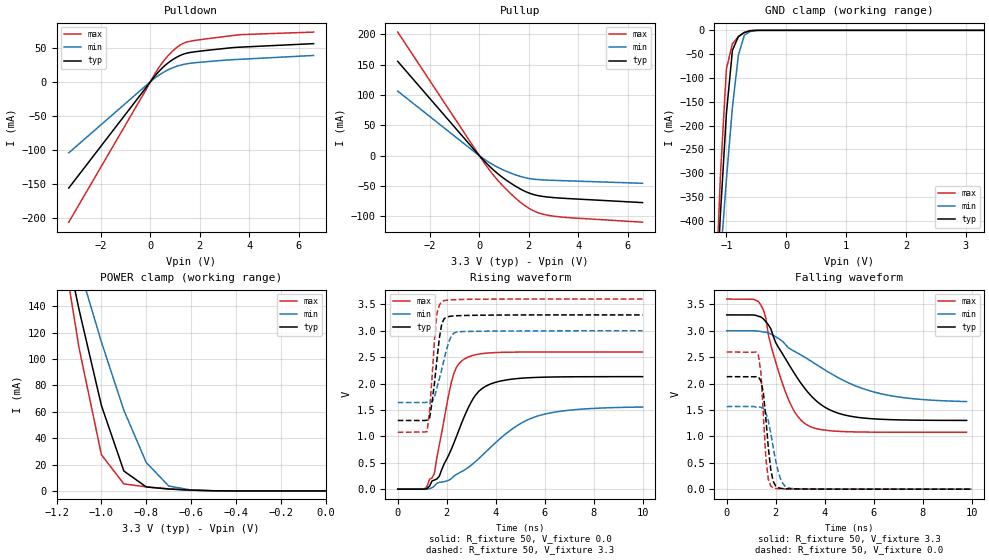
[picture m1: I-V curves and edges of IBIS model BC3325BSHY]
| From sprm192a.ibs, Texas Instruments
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[Model]   BC3325BSHY
Model_type   I/O
Vinh = 2.00
Vinl = 0.80
Enable   Active-Low
Polarity   Non-Inverting
| signals   A, GZ, Y
Vmeas = 1.5
|   typ   min   max
C_comp   1.4592p   1.4336p   1.5063p
|   typ   min   max
[Temperature Range]   25   -40   125
|   typ   min   max
[Voltage Range]   3.30V   3.00V   3.60V
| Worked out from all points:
|   slope of the pulldown table from 0 to 0.495 V, typ, clamps not added: 24 ohm
|   slope of the pullup table from 0 to 0.495 V, typ, clamps not added: 23.8 ohm
|   GND clamp passes 1 mA (typ) near -0.60 V on its own axis
|   POWER clamp passes 1 mA (typ) near -0.65 V on its own axis
|   rising waveform, R_fixture 50, V_fixture 0.0: 20-80 % time 1.22ns typ, 2.5ns min, 651ps max; typ from 0 V to 2.13 V
|   falling waveform, R_fixture 50, V_fixture 3.3: 20-80 % time 1.69ns typ, 3.01ns min, 992ps max; typ from 3.3 V to 1.3 V
|   rising waveform, R_fixture 50, V_fixture 3.3: 20-80 % time 298ps typ, 453ps min, 241ps max; typ from 1.3 V to 3.3 V
|   falling waveform, R_fixture 50, V_fixture 0.0: 20-80 % time 263ps typ, 401ps min, 201ps max; typ from 2.13 V to 0 V
[Pulldown]
|   Voltage   I(typ)   I(min)   I(max)
-3.3V     -155.6mA   -104.1mA   -205.7mA
200mV     9.245mA    5.867mA    12.7mA
600mV     24.13mA    15.28mA    33.3mA
800mV     29.87mA    18.87mA    41.37mA
1.1V      36.63mA    23.02mA    51.08mA
1.3V      39.97mA    25.04mA    55.82mA
1.6V      42.83mA    27mA       59.29mA
3.5V      50.44mA    32.65mA    68.4mA
6.6V      55.85mA    38.51mA    72.74mA
[GND_clamp]
|   Voltage   I(typ)   I(min)   I(max)
-3.3V     -6.256A    -4.713A    -8.133A
-1.2V     -625.1mA   -657.9mA   -612.5mA
-1.1V     -386.1mA   -480.8mA   -304.3mA
-1V       -174.5mA   -312.6mA   -80.61mA
-900mV    -42.06mA   -162mA     -28.39mA
-800mV    -12.94mA   -52.09mA   -13.55mA
-700mV    -4.666mA   -10.15mA   -3.941mA
-600mV    -901.9uA   -2.273mA   -447.8uA
-400mV    -4.618uA   -49.07uA   -472nA
3.3V      133.2pA    1.904uA    0A
[Pullup]
|   Voltage   I(typ)   I(min)   I(max)
-3.3V     155.5mA    106.5mA    203.8mA
-200mV    9.305mA    6.232mA    12.42mA
300mV     -13.07mA   -8.545mA   -17.75mA
600mV     -24.68mA   -16mA      -33.64mA
900mV     -34.78mA   -22.33mA   -47.63mA
1.4V      -48.81mA   -30.78mA   -67.77mA
1.7V      -55.89mA   -34.78mA   -78.18mA
2V        -61.53mA   -37.68mA   -86.7mA
2.3V      -65.31mA   -39.22mA   -93.01mA
2.9V      -68.84mA   -40.61mA   -99.22mA
3.7V      -71.03mA   -41.73mA   -102.5mA
6.6V      -77.47mA   -45.64mA   -109.8mA
[POWER_clamp]
|   Voltage   I(typ)   I(min)   I(max)
-3.3V     2.13A      1.607A     2.766A
-1.2V     219.2mA    230.5mA    214.4mA
-1.1V     137.7mA    170.3mA    108.7mA
-1V       64.77mA    112.9mA    27.43mA
-900mV    15.1mA     61.17mA    5.337mA
-800mV    3.01mA     21.5mA     3.051mA
-700mV    1.426mA    3.717mA    1.578mA
-600mV    596.1uA    671uA      553.1uA
0V        399.7pA    9.948nA    88.82pA
[Ramp]
|   I(typ)   I(min)   I(max)
dV/dt_r   1.278/1.224n   0.933/2.499n   1.559/0.649n
dV/dt_f   1.199/1.689n   0.806/3.020n   1.513/0.992n
[Rising Waveform]
R_fixture = 50
V_fixture = 0.0
|  pu_on
|  TIME   V(typ)   V(min)   V(max)
0s        3nV        16nV       2nV
1.1ns     -133.6uV   -280.8uV   2.733mV
1.4ns     153.6mV    26.81mV    210.9mV
1.5ns     172.7mV    58.73mV    301.8mV
2.2ns     766.4mV    203.2mV    2.04V
2.4ns     998.4mV    280.9mV    2.307V
2.8ns     1.46V      385.3mV    2.485V
3.6ns     1.95V      706.3mV    2.575V
5.6ns     2.115V     1.367V     2.597V
10ns      2.131V     1.554V     2.598V
[Falling Waveform]
R_fixture = 50
V_fixture = 3.3
V_fixture_min = 3.0
V_fixture_max = 3.6
|  pd_on
|  TIME   V(typ)   V(min)   V(max)
0s        3.3V       3V         3.6V
1.4ns     3.26V      2.985V     3.481V
1.8ns     3.038V     2.939V     2.735V
2.4ns     2.471V     2.74V      1.842V
2.8ns     2.168V     2.602V     1.445V
3.3ns     1.845V     2.467V     1.212V
4ns       1.555V     2.261V     1.119V
5ns       1.386V     2.009V     1.087V
6.9ns     1.314V     1.754V     1.078V
9.8ns     1.302V     1.659V     1.078V
[Rising Waveform]
R_fixture = 50
V_fixture = 3.3
V_fixture_min = 3.0
V_fixture_max = 3.6
|  pd_off
|  TIME   V(typ)   V(min)   V(max)
0s        1.301V     1.64V      1.078V
1.2ns     1.306V     1.646V     1.089V
1.3ns     1.343V     1.65V      1.497V
1.5ns     2.002V     1.743V     2.822V
1.6ns     2.442V     1.919V     3.318V
1.7ns     2.861V     2.089V     3.488V
1.8ns     3.134V     2.275V     3.552V
2.1ns     3.271V     2.805V     3.583V
2.4ns     3.284V     2.974V     3.589V
10ns      3.3V       3V         3.6V
[Falling Waveform]
R_fixture = 50
V_fixture = 0.0
|  pu_off
|  TIME   V(typ)   V(min)   V(max)
0s        2.131V     1.565V     2.598V
1.3ns     2.125V     1.554V     2.528V
1.4ns     2.046V     1.551V     2.202V
1.5ns     1.82V      1.526V     1.39V
1.6ns     1.34V      1.448V     585.8mV
1.7ns     789.5mV    1.294V     184.5mV
1.9ns     148.2mV    792.6mV    22.85mV
2.2ns     16mV       196mV      7.078mV
2.5ns     6.884mV    26.38mV    4.109mV
10ns      2.497uV    60.61uV    1.686uV
